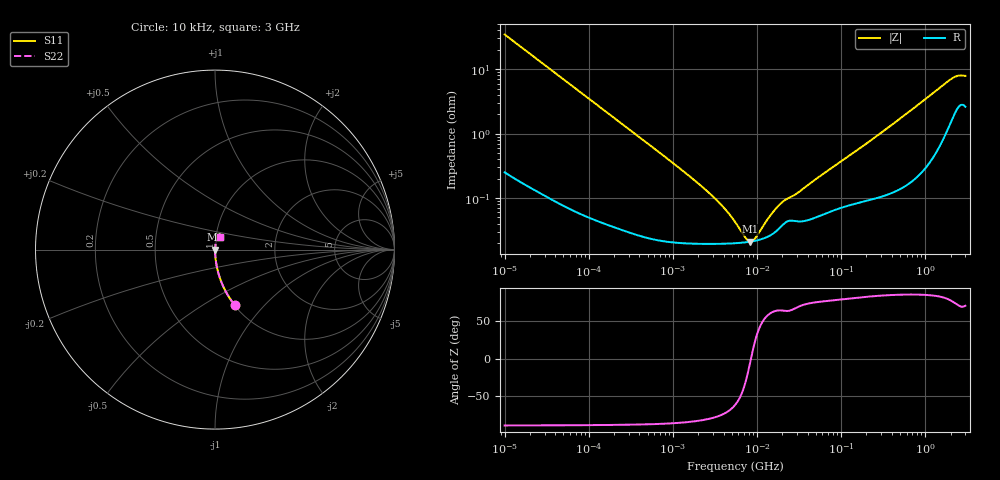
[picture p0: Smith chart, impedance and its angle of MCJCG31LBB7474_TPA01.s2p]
! MCJCG31LBB7474_TPA01  S-PARAMETER MODEL  ( Standard Model )
! Model Generated by TAIYO YUDEN Corporation (http://www.ty-top.com)
! Version 1.0
! TAIYO YUDEN Control No. 220601
! Copyright(c) 2015 TAIYO YUDEN CO.,LTD. All Rights Reserved.
! Product Description (link to TY-COMPAS)
! https://ds.yuden.co.jp/TYCOMPAS/or/detail?pn=MCJCG31LBB7474KTPA01&u=M
! Products Name : Multilayer Ceramic Capacitors
! Characteristics :
!  Capacitance : 0.47 [uF] , Rated Voltage : 35 [V] , TCC : X7R
!  Case Size : 3.2 x 1.6 / 0.126 x 0.063 [mm/inch] , Thickness : 1.6 / 0.063 [mm/inch]
!  (Conditions: Temperature = 25 [degC] , DC Bias Voltage = 0 [V])
! External Node Assignments :
!  1  o---| |---o  2
! GND o---------o GND
! Frequency Range : 10kHz  -  3GHz  [ 401 STEP ]
# MHZ S RI R 50
! Freq[MHz].  S11 Real  S11 Imag  S21 Real  S21 Imag  S12 Real  S12 Imag  S22 Real  S22 Imag
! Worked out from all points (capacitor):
!   401 points, 10 kHz to 3 GHz, reference 50 ohm
!   read as one part in series: C = 459 nF near 10.65 kHz
!   lowest |Z| = 21.1 mohm at 8.252 MHz (marker M1)
!   series resonance near 8.487 MHz, so ESL is about 770 pH
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0.01  0.1089 -0.3079  0.8911 0.3079  0.8911 0.3079  0.1089 -0.3079
0.015549  0.049 -0.2119  0.951 0.2119  0.951 0.2119  0.049 -0.2119
0.026575  0.018 -0.1284  0.982 0.1284  0.982 0.1284  0.018 -0.1284
0.082683  0.00234 -0.0422  0.9977 0.0422  0.9977 0.0422  0.00234 -0.0422
0.683653  0.000246 -0.00515  0.9998 0.00515  0.9998 0.00515  0.000246 -0.00515
1.601553  0.000201 -0.00214  0.9998 0.00214  0.9998 0.00214  0.000201 -0.00214
2.737278  0.000195 -0.00116  0.9998 0.00116  0.9998 0.00116  0.000195 -0.00116
3.996065  0.000196 -0.000692  0.9998 0.000692  0.9998 0.000692  0.000196 -0.000692
5.477226  0.000199 -0.000379  0.9998 0.000379  0.9998 0.000379  0.000199 -0.000379
7.274378  0.000205 -0.00013  0.9998 0.00013  0.9998 0.00013  0.000205 -0.00013
8.252149  0.00021 -2.35e-05  0.9998 2.35e-05  0.9998 2.35e-05  0.00021 -2.35e-05
8.789267  0.000213 2.95e-05  0.9998 -2.95e-05  0.9998 -2.95e-05  0.000213 2.95e-05
9.6612  0.000218 0.000109  0.9998 -0.000109  0.9998 -0.000109  0.000218 0.000109
14.10408  0.00026 0.000447  0.9997 -0.000447  0.9997 -0.000447  0.00026 0.000447
18.73182  0.000346 0.000723  0.9997 -0.000723  0.9997 -0.000723  0.000346 0.000723
21.93027  0.000419 0.000847  0.9996 -0.000847  0.9996 -0.000847  0.000419 0.000847
30.05882  0.000436 0.00111  0.9996 -0.00111  0.9996 -0.00111  0.000436 0.00111
45.28751  0.000479 0.00172  0.9995 -0.00172  0.9995 -0.00172  0.000479 0.00172
374.4521  0.00132 0.0128  0.9987 -0.0128  0.9987 -0.0128  0.00132 0.0128
1991.2  0.0187 0.0656  0.9813 -0.0656  0.9813 -0.0656  0.0187 0.0656
2405.867  0.029 0.071  0.971 -0.071  0.971 -0.071  0.029 0.071
3000  0.0306 0.0704  0.9694 -0.0704  0.9694 -0.0704  0.0306 0.0704
